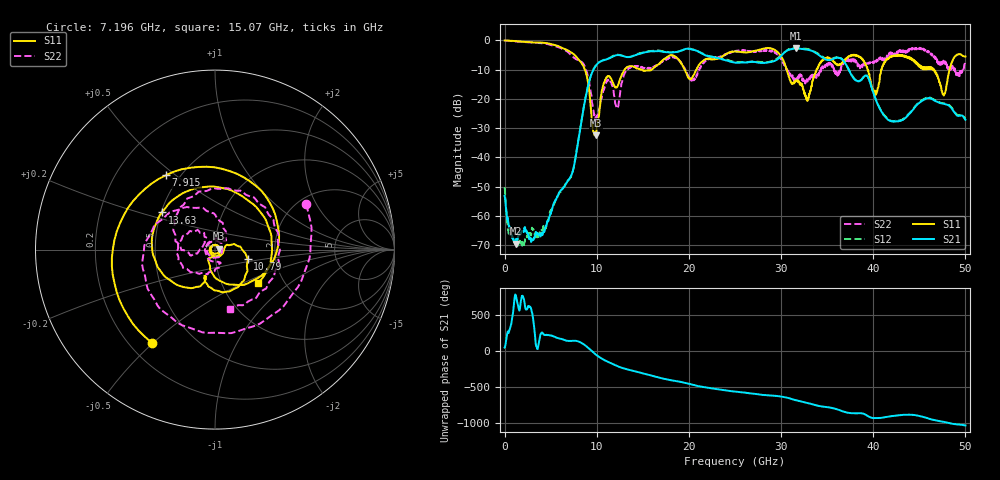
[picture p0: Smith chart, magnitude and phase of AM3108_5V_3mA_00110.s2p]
# Hz S DB R 50.0
!freq dBS11 angS11 dBS21 angS21 dBS12 angS12 dBS22 angS22
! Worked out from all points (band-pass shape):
!   1601 points, 10 MHz to 50 GHz, reference 50 ohm
!   highest |S21| = -2.75 dB at 31.66 GHz (marker M1); lowest = -69.5 dB at 1.197 GHz (marker M2)
!   |S21| within 3 dB of the highest: 11.59 GHz to 22.75 GHz (11.16 GHz wide, 65 % of centre); 29.87 GHz to 34.45 GHz (4.573 GHz wide, 14.2 % of centre)
!   lowest |S11| = -32.5 dB at 9.883 GHz (marker M3), VSWR 1.05, Z = 52.4 + j0.552 ohm
!   |S11| at or under -10 dB: 8.72 GHz to 13.02 GHz (4.297 GHz wide, 39.5 % of centre); 30.63 GHz to 33.85 GHz (3.22 GHz wide, 9.99 % of centre); 46.62 GHz to 48.29 GHz (1.666 GHz wide, 3.51 % of centre)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
!   |S22| runs from -27.6 to 0.0 dB; largest |S21 - S12| = 0.025
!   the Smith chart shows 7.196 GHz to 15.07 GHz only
!   S11 on the Smith chart (normalised r, x): 7.196 GHz: 0.29, -0.50; 7.915 GHz: 0.42, +0.46; 10.79 GHz: 1.43, -0.16; 13.63 GHz: 0.50, +0.24; 15.07 GHz: 1.48, -0.61
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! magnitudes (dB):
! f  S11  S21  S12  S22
! 10 MHz  0.0  -53.1  -50.2  0.0
! 1.197 GHz  -0.2  -69.5  -69.3  -0.3
! 4.103 GHz  -0.8  -66.6  -65.0  -1.0
! 7.196 GHz  -4.0  -46.5  -46.8  -4.9
! 7.915 GHz  -6.1  -36.1  -35.9  -6.6
! 8.352 GHz  -7.7  -27.4  -27.3  -7.3
! 9.883 GHz  -32.5  -8.8  -8.7  -26.3
! 10.79 GHz  -14.5  -6.8  -6.6  -16.8
! 12.23 GHz  -15.9  -5.0  -4.9  -23.2
! 13.63 GHz  -8.8  -5.6  -5.6  -9.2
! 15.07 GHz  -10.4  -4.2  -4.1  -9.4
! 16.69 GHz  -8.2  -3.6  -3.4  -8.4
! 20.41 GHz  -12.4  -3.2  -3.0  -13.8
! 25 GHz  -3.8  -7.6  -7.4  -3.8
! 29.16 GHz  -3.0  -7.2  -6.9  -3.7
! 31.66 GHz  -13.9  -2.8  -2.7  -13.9
! 33.35 GHz  -15.4  -3.6  -3.4  -12.7
! 38 GHz  -4.9  -13.4  -13.3  -6.6
! 40.22 GHz  -18.9  -19.8  -19.7  -7.6
! 41.69 GHz  -6.0  -27.3  -27.1  -5.2
! 47.66 GHz  -18.8  -21.7  -21.6  -7.7
! 50 GHz  -5.5  -27.1  -26.6  -6.8
